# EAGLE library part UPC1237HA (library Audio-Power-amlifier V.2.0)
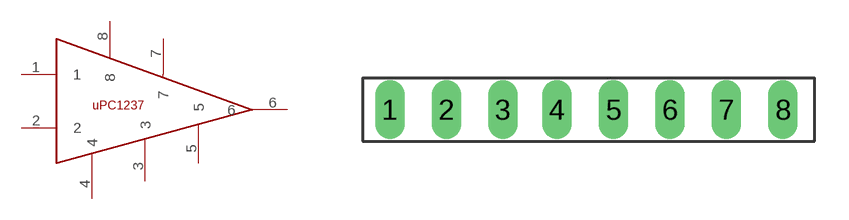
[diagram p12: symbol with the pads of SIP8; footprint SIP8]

Designator prefix U

## UPC1237HA  [SIP8]
1  1
2  2
3  3
4  4
5  5
6  6
7  7
8  8

## Footprint SIP8 (pad centres in mm)
drill 0.8 long: 1 -8.8,3.6; 2 -6.3,3.6; 3 -3.8,3.6; 4 -1.4,3.6; 5 1.1,3.6; 6 3.6,3.6; 7 6.1,3.6; 8 8.6,3.6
